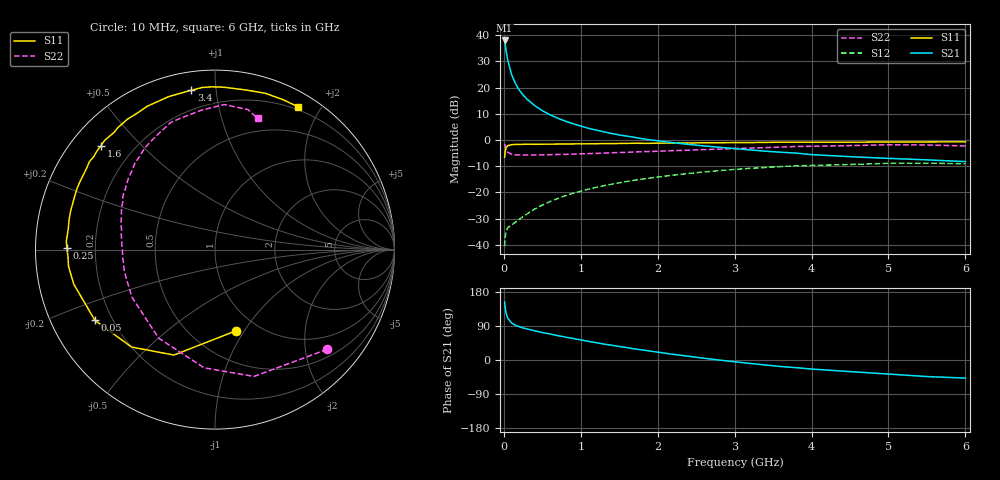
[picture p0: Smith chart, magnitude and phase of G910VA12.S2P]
! SIEMENS Small Signal Semiconductors
! BFG235
! Si NPN RF Bipolar Junction Transistor in SOT223
! VCE = 10 V  IC = 120 mA
! Common Emitter S-Parameters:  July  1994
# GHz  S  MA  R  50
!  f  S11  S21  S12  S22
! GHz  MAG  ANG  MAG  ANG  MAG  ANG  MAG  ANG
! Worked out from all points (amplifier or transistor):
!   40 points, 10 MHz to 6 GHz, reference 50 ohm
!   highest |S21| = 38.0 dB at 10 MHz (marker M1)
!   |S21| within 3 dB of that: start of sweep to 25.1 MHz
!   unconditionally stable (mu >= 1): 475.3 MHz to 1.477 GHz
!   at 200 MHz: K = 0.77, MSG = 24.7 dB, |S12| = -30.3 dB
!   at 1.5 GHz: K = 1.00, MSG = 9.1 dB, |S12| = -16.4 dB
!   at 6 GHz: K = 0.90, MSG = 0.4 dB, |S12| = -9.1 dB
!   S11 on the Smith chart (normalised r, x): 10 MHz: 0.79, -0.92; 50 MHz: 0.14, -0.27; 250 MHz: 0.10, +0.01; 1.6 GHz: 0.09, +0.39; 3.4 GHz: 0.09, +0.86; 6 GHz: 0.17, +1.73
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0.01  0.4677 -75.8  79.2 153.5  0.0094 64.3  0.8364 -41.6
0.02  0.6306 -111.3  63.16 134.9  0.0148 50.8  0.7393 -72.9
0.03  0.7148 -130.6  50.01 123.1  0.018 41.9  0.6614 -95.3
0.05  0.7765 -149.5  33.56 110.2  0.0211 33.9  0.5847 -122.5
0.1  0.8102 -166.3  17.81 97.8  0.0239 35.4  0.5333 -150.0
0.15  0.8213 -173.5  11.99 91.8  0.0268 41.0  0.52 -161.4
0.2  0.82 -177.3  8.966 87.9  0.0307 45.4  0.5187 -167.6
0.25  0.8255 179.3  7.222 84.6  0.0344 49.8  0.5155 -171.8
0.3  0.8297 176.8  6.03 82.0  0.0385 52.6  0.5163 -175.1
0.4  0.8255 172.2  4.534 77.0  0.048 56.3  0.516 -179.6
0.5  0.8298 168.4  3.623 72.5  0.0572 58.3  0.52 176.9
0.6  0.8324 165.2  3.025 68.7  0.0665 58.9  0.5237 173.8
0.7  0.8338 161.7  2.603 64.3  0.0766 59.2  0.5285 171.0
0.9  0.8409 156.2  2.038 56.8  0.0958 57.7  0.5367 166.5
1.1  0.8441 149.8  1.67 49.1  0.115 55.4  0.5495 162.0
1.6  0.8598 137.6  1.182 32.7  0.1617 47.7  0.5805 152.0
2.2  0.875 124.0  0.887 15.0  0.2128 37.2  0.6256 140.4
3.2  0.892 102.7  0.646 -9.1  0.2871 17.9  0.6986 121.4
3.4  0.8978 98.4  0.61 -13.1  0.2986 13.8  0.7139 117.1
4.5  0.9059 79.0  0.48 -30.6  0.341 -7.2  0.7796 95.8
5.5  0.9173 65.5  0.417 -43.7  0.3613 -25.8  0.8014 76.8
6  0.9204 59.7  0.386 -47.7  0.3511 -32.6  0.7688 72.0
